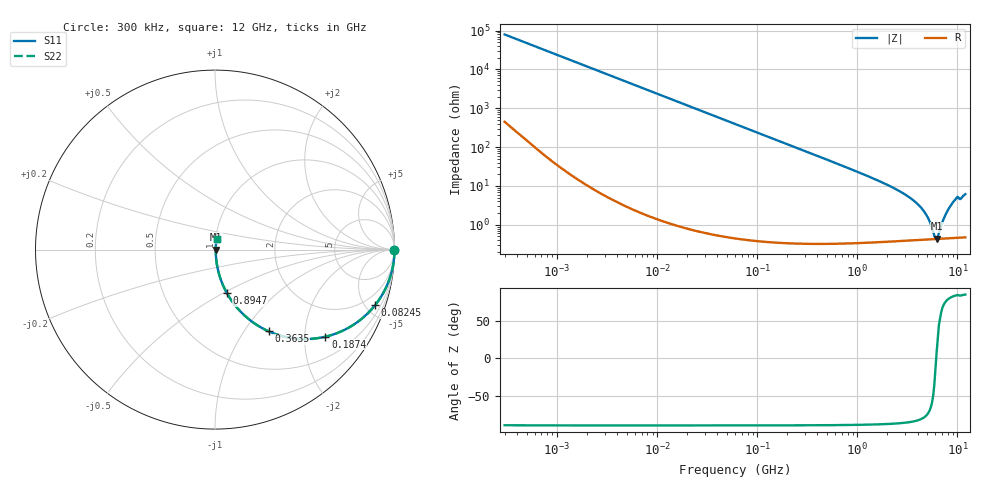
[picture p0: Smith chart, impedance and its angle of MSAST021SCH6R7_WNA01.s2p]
! MSAST021SCH6R7_WNA01  S-PARAMETER MODEL  ( General Type )
! Model Generated by TAIYO YUDEN Corporation (http://www.ty-top.com)
! Version 2.0
! TAIYO YUDEN Control No. 181101
! Copyright(c) 2015 TAIYO YUDEN CO.,LTD. All Rights Reserved.
! Product Description (link to TY-COMPAS)
! https://ds.yuden.co.jp/TYCOMPAS/or/detail?pn=MSAST021SCH6R7CWNA01&u=M
! Products Name : Multilayer Ceramic Capacitors
! Characteristics :
!  Capacitance : 6.7 pF , Rated Voltage : 25V , TCC : CH / C0H
!  Case Size : 0.25 x 0.125 / 0.0098 x 0.0049 [mm/inch] , Thickness : 0.125 / 0.0049 [mm/inch]
!  (Conditions: Temperature = 25 degC , DC Bias Current/Voltage = 0A / 0V)
! External Node Assignments :
!  1  o---| |---o  2
! GND o---------o GND
! Frequency Range : 0.3MHz  -  12000MHz  [ 401 STEP ]
# MHz S RI R 50
! Freq[MHz].  S11 Real  S11 Imag  S21 Real  S21 Imag  S12 Real  S12 Imag  S22 Real  S22 Imag
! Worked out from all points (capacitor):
!   401 points, 300 kHz to 12 GHz, reference 50 ohm
!   read as one part in series: C = 6.7 pF near 316.3 kHz
!   lowest |Z| = 436 mohm at 6.188 GHz (marker M1)
!   series resonance near 6.132 GHz, so ESL is about 100 pH
!   S11 on the Smith chart (normalised r, x): 300 kHz: open; 82.45 MHz: 1.01, -5.76; 187.4 MHz: 1.01, -2.53; 363.5 MHz: 1.01, -1.30; 894.7 MHz: 1.01, -0.52; 12 GHz: 1.01, +0.12
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0.3  1 -0.00126  8.74e-06 0.00126  8.74e-06 0.00126  1 -0.00126
1.769972  0.9999 -0.00745  6.25e-05 0.00745  6.25e-05 0.00745  0.9999 -0.00745
10.44266  0.998 -0.0439  0.00195 0.0439  0.00195 0.0439  0.998 -0.0439
27.10171  0.9871 -0.1126  0.0129 0.1126  0.0129 0.1126  0.9871 -0.1126
60  0.9398 -0.2373  0.0602 0.2373  0.0602 0.2373  0.9398 -0.2373
82.45425  0.8921 -0.3096  0.1079 0.3096  0.1079 0.3096  0.8921 -0.3096
187.4445  0.6155 -0.4851  0.3845 0.4851  0.3845 0.4851  0.6155 -0.4851
353.9943  0.3099 -0.4601  0.6901 0.4601  0.6901 0.4601  0.3099 -0.4601
363.4975  0.2987 -0.4552  0.7013 0.4552  0.7013 0.4552  0.2987 -0.4552
555.3718  0.1544 -0.3575  0.8456 0.3575  0.8456 0.3575  0.1544 -0.3575
894.6982  0.066 -0.2419  0.934 0.2419  0.934 0.2419  0.066 -0.2419
2088.533  0.0135 -0.0987  0.9865 0.0987  0.9865 0.0987  0.0135 -0.0987
3107.553  0.00705 -0.056  0.993 0.056  0.993 0.056  0.00705 -0.056
4158.869  0.00499 -0.0304  0.995 0.0304  0.995 0.0304  0.00499 -0.0304
5006.236  0.00441 -0.0154  0.9956 0.0154  0.9956 0.0154  0.00441 -0.0154
5868.704  0.00428 -0.00309  0.9957 0.00309  0.9957 0.00309  0.00428 -0.00309
6188.031  0.00431 0.000554  0.9957 -0.000554  0.9957 -0.000554  0.00431 0.000554
6524.734  0.00436 0.00426  0.9956 -0.00426  0.9956 -0.00426  0.00436 0.00426
7648.807  0.00477 0.0182  0.9952 -0.0182  0.9952 -0.0182  0.00477 0.0182
8732.115  0.00561 0.0328  0.9944 -0.0328  0.9944 -0.0328  0.00561 0.0328
9708.23  0.00681 0.0469  0.9932 -0.0469  0.9932 -0.0469  0.00681 0.0469
12000  0.00841 0.0604  0.9916 -0.0604  0.9916 -0.0604  0.00841 0.0604
